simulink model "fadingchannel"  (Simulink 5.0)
settings: Solver=ode5  StartTime=0.0  StopTime=5  RelTol=1e-3
libraries: dspxfrm3 x1, commnoisgen2 x1, dspstat3 x1, simulink x1, commchan2 x1

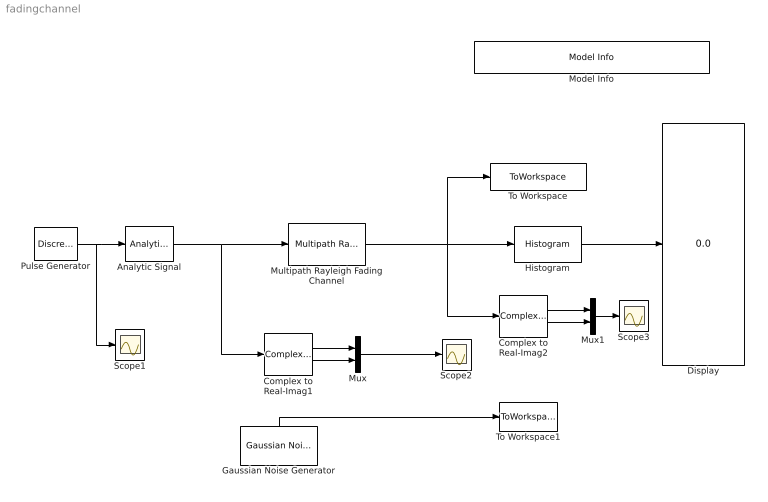
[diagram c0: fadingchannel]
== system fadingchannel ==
  Analytic Signal : dspxfrm3/Analytic Signal  N=100
  Complex to Real-Imag1 : ComplexToRealImag
  Complex to Real-Imag2 : ComplexToRealImag
  Display : Display
  Gaussian Noise Generator : commnoisgen2/Gaussian Noise Generator  Orientation=up  m=0  d=1  s=41  Ts=.0001  frameBased=off  sampPerFrame=1  orient=off
  Histogram : dspstat3/Histogram  umin=-1.45  umax=1.45  nbins=13  normalized=on  run=on  reset=off  trigtype=Either edge
  Model Info : simulink/Model-Wide Utilities/Model Info  InitialBlockCM=None  BlockCM=None  Frame=on  DisplayStringWithTags=Rayleigh Fading Channel  HorizontalTextAlignment=Center  LeftAlignmentValue=0.5  SourceBlockDiagram=fadingchannel  TagMaxNumber=20
  Multipath Rayleigh Fading Channel : commchan2/Multipath Rayleigh Fading Channel  Fd=40  simTs=1e-4  delayVec=[0 2e-6]  gainVecdB=[0 -3]  normGain=on  Seed=73
  Mux : Mux  Inputs=2
  Mux1 : Mux  Inputs=2
  Pulse Generator : DiscretePulseGenerator  SampleTime=.0001
  Scope1 : Scope
  Scope2 : Scope
  Scope3 : Scope
  To Workspace : ToWorkspace  VariableName=RayleighPDFOutput  SampleTime=-1  SaveFormat=Structure
  To Workspace1 : ToWorkspace  VariableName=AWGN  SampleTime=-1  SaveFormat=Structure
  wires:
  Complex to Real-Imag1/1 -> Mux/1
  Complex to Real-Imag1/2 -> Mux/2
  Mux/1 -> Scope2/1
  Complex to Real-Imag2/1 -> Mux1/1
  Complex to Real-Imag2/2 -> Mux1/2
  Mux1/1 -> Scope3/1
  Pulse Generator/1 -> Analytic Signal/1, Scope1/1
  Analytic Signal/1 -> Multipath Rayleigh Fading Channel/1, Complex to Real-Imag1/1
  Multipath Rayleigh Fading Channel/1 -> Complex to Real-Imag2/1, To Workspace/1, Histogram/1
  Histogram/1 -> Display/1
  Gaussian Noise Generator/1 -> To Workspace1/1
